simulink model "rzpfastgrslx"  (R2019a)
settings: configuration reference "configurationSettings" (kept in a data dictionary, not in this file)
model workspace (MATLAB code in the model file):
  other statements: [L,TP] = rzpfastgrslx_init();
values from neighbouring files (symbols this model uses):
  L = fbtc(P,G)    [fbt.m]    (also in fbtc.m = meqc(P,G); fbte.m = varargout{1})
undefined symbols (not defined in the file or in its folder): TP

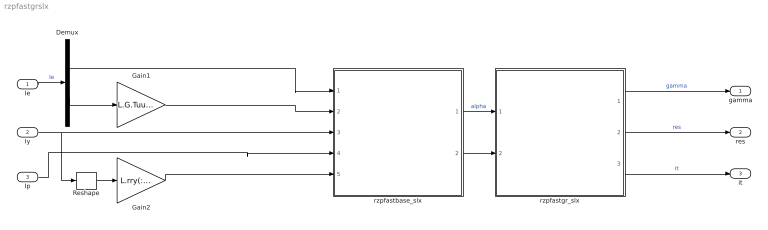
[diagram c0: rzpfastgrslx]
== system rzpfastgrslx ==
  Ie : Inport  OutDataTypeStr=single  Interpolate=off
  Iy : Inport  Port=2  OutDataTypeStr=single  Interpolate=off
  Ip : Inport  Port=3  OutDataTypeStr=single  Interpolate=off
  Demux : Demux  Outputs=2
  Gain1 : Gain  Gain=L.G.Tuuliu  Multiplication=Matrix(K*u) (u vector)
  Gain2 : Gain  Gain=L.rry(:)'  Multiplication=Matrix(K*u) (u vector)
  Reshape : Reshape
  rzpfastbase_slx : MATLAB Function  TreatAsAtomicUnit=on  mask{F=L.F, N=L.N, Trd=L.Trd, Tzd=L.Tzd, ny=L.ny, np=L.np, ne=L.ne, RBrye=L.RBrye, RBzye=L.RBzye, RBrye_fast=L.RBrye_fast, RBzye_fast=L.RBzye_fast}
  rzpfastgr_slx : MATLAB Function  TreatAsAtomicUnit=on  mask{dd=L.dd, dmax=L.dmax, iter_max=TP.iter_max, tol=TP.tol}
  gamma : Outport  SignalName=gamma
  res : Outport  Port=2  SignalName=res
  it : Outport  Port=3  SignalName=it
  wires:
  rzpfastgr_slx/1(gamma) -> gamma/1  "gamma"
  Ip/1 -> rzpfastbase_slx/4(Ip)
  rzpfastbase_slx/1(alpha) -> rzpfastgr_slx/1(alpha)  "alpha"
  Reshape/1 -> Gain2/1
  Iy/1 -> rzpfastbase_slx/3(Iy), Reshape/1
  rzpfastbase_slx/2(c) -> rzpfastgr_slx/2(c)
  rzpfastgr_slx/2(res) -> res/1  "res"
  rzpfastgr_slx/3(it) -> it/1  "it"
  Gain1/1 -> rzpfastbase_slx/2(Iu)
  Gain2/1 -> rzpfastbase_slx/5(rIp)
  Demux/1 -> rzpfastbase_slx/1(Ia)
  Ie/1 -> Demux/1  "Ie"
  Demux/2 -> Gain1/1

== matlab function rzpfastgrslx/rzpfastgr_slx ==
function [gamma,res,it] = rzpfastgr_slx(alpha,c,dd,dmax,iter_max, tol)

[gamma,res,it] = rzpfastgr(alpha,c,dd,dmax,iter_max,tol);

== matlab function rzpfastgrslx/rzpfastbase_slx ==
function [alpha,c] = rzpfastbase_slx(Ia,Iu,Iy,Ip,rIp,...
  N,F, Trd, Tzd, ny, np, ne, RBrye, RBzye, RBrye_fast, RBzye_fast)

[~,~,alpha,~,c] = rzpfastbase(Ia,Iu,Iy,Ip,rIp,...
  N,F,Trd,Tzd,ny,np,ne,RBrye,RBzye,RBrye_fast,RBzye_fast);
